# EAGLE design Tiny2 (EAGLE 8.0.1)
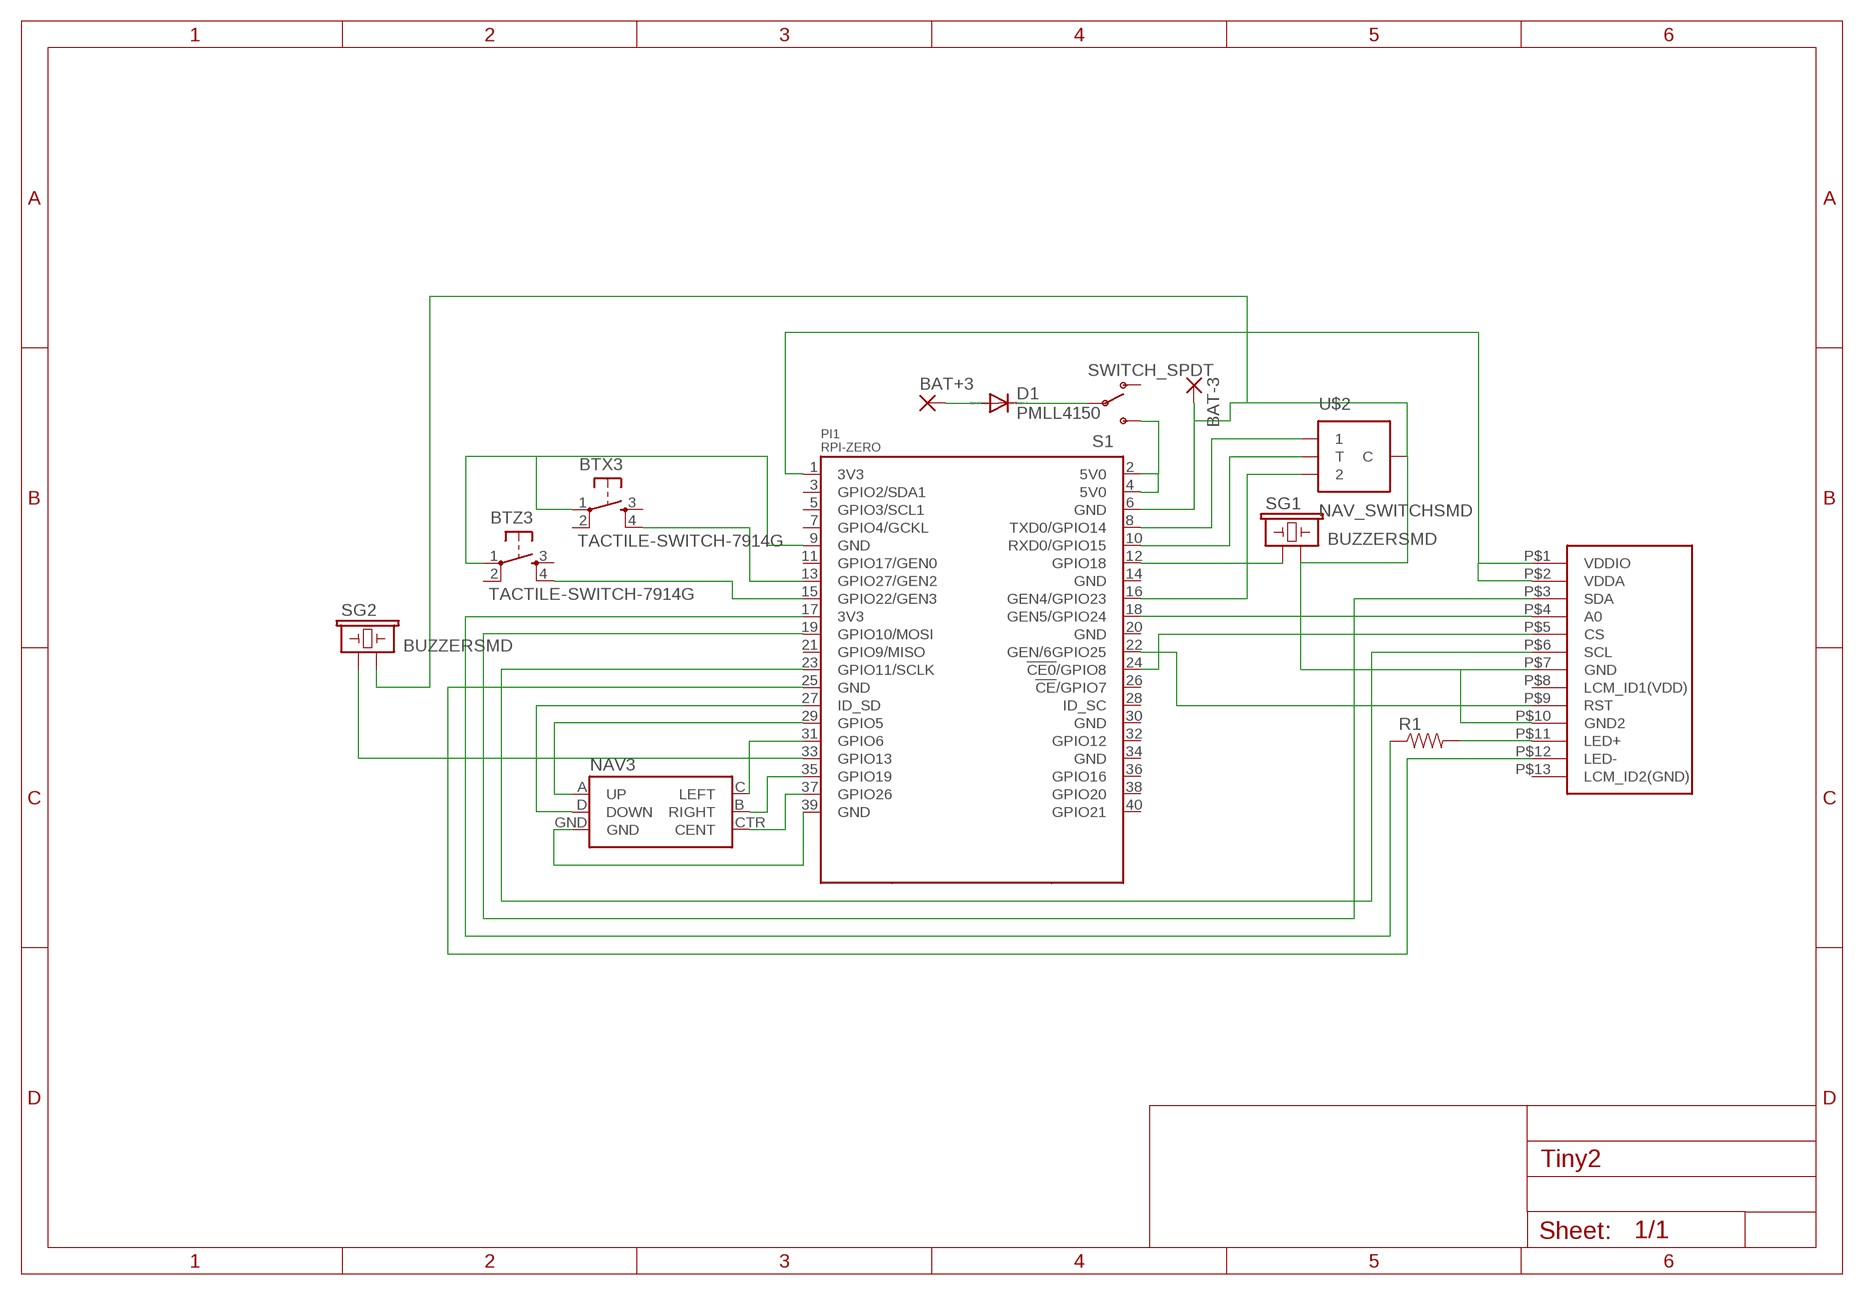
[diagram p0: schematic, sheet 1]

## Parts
BAT+3  SMD5  [SMD2,54-5,08]
BAT-3  SMD5  [SMD2,54-5,08]
BTX3  TACTILE-SWITCH-7914G  [7914G]
BTZ3  TACTILE-SWITCH-7914G  [7914G]
D1  PMLL4150  [SOD80C]
NAV3  JOYSTICK_MINI  [JOYSTICK_MINI]
PI1  RPI-ZERO  [RASPBERRYPI_BASTELSTUBE_V13_RASPI_BOARD_B+_FULL]
R1  RESISTOR0805-RES  [0805]
S1  SWITCH_SPDT  [KPS-1290]
SG1  BUZZERSMD  [BUZZER-CMT1603]
SG2  BUZZERSMD  [BUZZER-CMT1603]
U$1  ST7735S-1.44  [ST7735S-1.44]
U$2  NAV_SWITCHSMD  [NAV_SWITCH]

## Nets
3V3@1: PI1.1(3V3) U$1.P$1(VDDIO) U$1.P$2(VDDA)
3V3@2: PI1.17(3V3) R1.1
5V0@2: PI1.2(5V0) PI1.4(5V0) S1.S
GND@1: BTX3.1 BTZ3.1 PI1.9(GND)
GND@2: PI1.25(GND) U$1.P$12(LED-)
GND@3: NAV3.GND PI1.39(GND)
GND@8: BAT-3.1(P) PI1.6(GND) SG1.P$2 SG2.P$2 U$1.P$7(GND) U$1.P$10(GND2) U$2.C
N$1: PI1.22(GEN/6GPIO25) U$1.P$9(RST)
N$2: PI1.23(GPIO11/SCLK) U$1.P$6(SCL)
N$3: PI1.19(GPIO10/MOSI) U$1.P$3(SDA)
N$4: NAV3.CTR(CENT) PI1.37(GPIO26)
N$5: NAV3.B(RIGHT) PI1.35(GPIO19)
N$6: PI1.18(GEN5/GPIO24) U$1.P$4(A0)
N$7: PI1.24(!CE0!/GPIO8) U$1.P$5(CS)
N$8: NAV3.C(LEFT) PI1.31(GPIO6)
N$9: NAV3.A(UP) PI1.29(GPIO5)
N$10: NAV3.D(DOWN) PI1.27(ID_SD)
N$11: BTZ3.4 PI1.15(GPIO22/GEN3)
N$12: BTX3.4 PI1.13(GPIO27/GEN2)
N$13: PI1.12(GPIO18) SG1.P$1
N$14: R1.2 U$1.P$11(LED+)
N$15: PI1.33(GPIO13) SG2.P$1
N$16: PI1.8(TXD0/GPIO14) U$2.1
N$17: PI1.10(RXD0/GPIO15) U$2.T
N$18: PI1.16(GEN4/GPIO23) U$2.2
N$20: BAT+3.1(P) D1.A
N$21: D1.C S1.P
Unconnected: BTX3.2 BTX3.3 BTZ3.2 BTZ3.3 PI1.3(GPIO2/SDA1) PI1.5(GPIO3/SCL1) PI1.7(GPIO4/GCKL) PI1.11(GPIO17/GEN0) PI1.14(GND) PI1.20(GND) PI1.21(GPIO9/MISO) PI1.26(!CE!/GPIO7) PI1.28(ID_SC) PI1.30(GND) PI1.32(GPIO12) PI1.34(GND) PI1.36(GPIO16) PI1.38(GPIO20) PI1.40(GPIO21) S1.O U$1.P$8(LCM_ID1(VDD)) U$1.P$13(LCM_ID2(GND))

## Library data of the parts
BAT+3 BAT-3 = wirepad:SMD5: SMD PAD
BTX3 BTZ3 = GeekAmmo:TACTILE-SWITCH: Tactile Switch 4 Pins, SPST NO
D1 = diode:PMLL4150: DIODE
NAV3 = SparkFun-Electromechanical:JOYSTICK_MINI: Small 5-way tactile joystick, COM-10063 4UCON SF303GJ26; PROD_ID: SWCH-09905
PI1 = RPI-Zero:RPI-ZERO
R1 = SparkFun-Resistors:RESISTOR: Resistor
S1 = SparkFun-Electromechanical:SWITCH_SPDT: SWCH-10651 Side-actuated SPDT slide switch, as used on the Arduino Pro; PROD_ID: SWCH-10651
SG1 SG2 = SparkFun-Electromechanical:BUZZER: Buzzer 12mm
U$1 = ST7735S:ST7735S-1.44
U$2 = SparkFun-Electromechanical:NAV_SWITCH: Navigation Switch Three way navigation switch. Commonly used as up/down/select on MP3 players. Schematic element and footprint production proven. Spark Fun Electronics SKU : COM-08184; PROD_ID: SWCH-08301

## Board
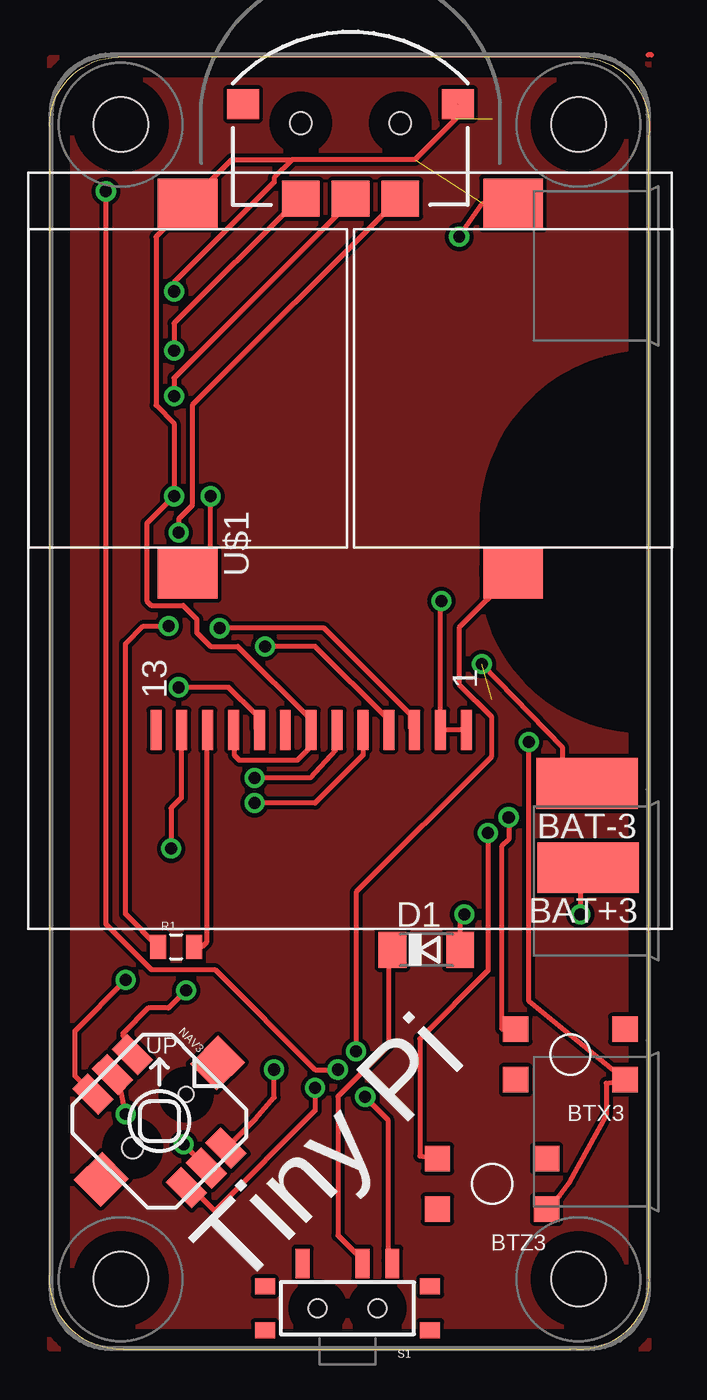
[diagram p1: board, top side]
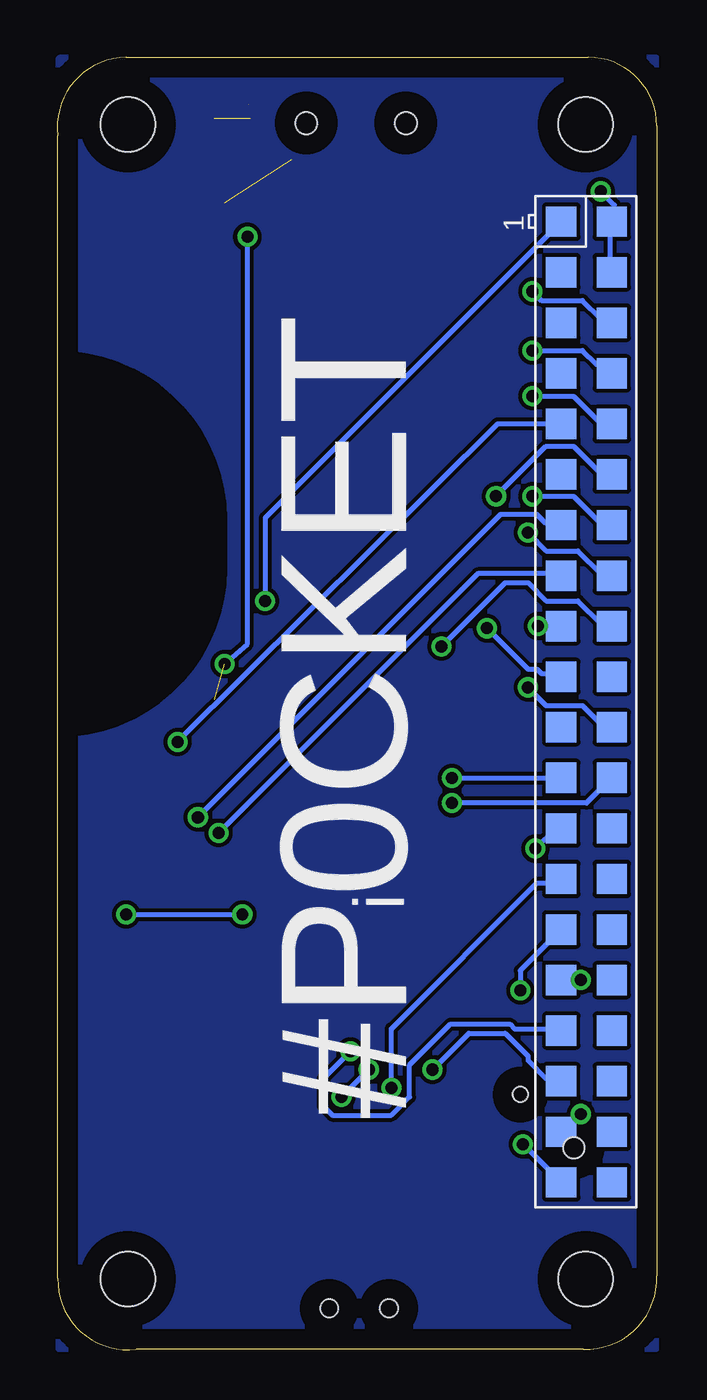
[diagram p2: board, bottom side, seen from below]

Size 30.12 x 64.92 mm. Coordinates in mm from the lower left corner, seen from the top.
Outline: 3.68,0.03 26.16,0.03 arc98 30.1,3.58 30.1,60.99 arc96 26.67,64.92 3.43,64.92 arc90 0,61.49 0,3.71 arc94 3.68,0.03
Copper layers (1*16): Top 0.035mm / dielectric 1.5mm / Bottom 0.035mm
Design rules "default *": minimum track width 10mil, minimum drill 24mil, track to track 8mil, track to pad 8mil, pad to pad 8mil, via to via 8mil, smd to smd 8mil, copper to edge 40mil, drill to drill 8mil, minimum pad ring 10mil, minimum via ring 8mil, stop-mask expansion 4mil, vias tented up to drill 25mil, thermal gap 10mil

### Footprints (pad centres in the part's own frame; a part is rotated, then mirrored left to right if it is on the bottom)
SMD2,54-5,08 = smd 2.54 x 5.08: 1 0,0
7914G = smd 1.27 x 1.27: 1 0,0; 2 0,5.486; 3 2.54,0; 4 2.54,5.486
SOD80C = smd 1.4 x 1.8: A 1.7,0; C -1.7,0
JOYSTICK_MINI = smd 1.85 x 1.1: A -3.325,1.4; B 3.325,1.4; C -3.325,-1.4; CTR -3.325,0; D 3.325,-1.4; GND 3.325,0 | smd 1.9 x 2: NC 0,4.13; NC@0 0,-4.13 | hole 0.75: 0,1.9 | hole 1.05: 0,-1.9
RASPBERRYPI_BASTELSTUBE_V13_RASPI_BOARD_B+_FULL = smd 1.524 x 1.524: 1 8.382,25.273; 2 8.382,27.813; 3 10.922,25.273; 4 10.922,27.813; 5 13.462,25.273; 6 13.462,27.813; 7 16.002,25.273; 8 16.002,27.813; 9 18.542,25.273; 10 18.542,27.813; 11 21.082,25.273; 12 21.082,27.813; 13 23.622,25.273; 14 23.622,27.813; 15 26.162,25.273; 16 26.162,27.813; 17 28.702,25.273; 18 28.702,27.813; 19 31.242,25.273; 20 31.242,27.813; 21 33.782,25.273; 22 33.782,27.813; 23 36.322,25.273; 24 36.322,27.813; 25 38.862,25.273; 26 38.862,27.813; 27 41.402,25.273; 28 41.402,27.813; 29 43.942,25.273; 30 43.942,27.813; 31 46.482,25.273; 32 46.482,27.813; 33 49.022,25.273; 34 49.022,27.813; 35 51.562,25.273; 36 51.562,27.813; 37 54.102,25.273; 38 54.102,27.813; 39 56.642,25.273; 40 56.642,27.813 | hole 2.75: 3.5,3.5; 3.5,26.5; 61.5,3.5; 61.5,26.5
0805 = smd 0.8 x 1.2: 1 -0.9,0; 2 0.9,0
KPS-1290 = smd 0.7 x 1.5: O -2.25,2.25; P 0.75,2.25; S 2.25,2.25 | smd 1 x 0.8: P$1 -4.15,1.1; P$2 -4.15,-1.1; P$3 4.15,-1.1; P$4 4.15,1.1 | hole 0.9: -1.5,0; 1.5,0
BUZZER-CMT1603 = smd 2.5 x 3: P$1 -9.3,0; P$2 9.3,0
ST7735S-1.44 = smd 2 x 0.55: P$1 -9,-5.85; P$2 -9,-4.55; P$3 -9,-3.25; P$4 -9,-1.95; P$5 -9,-0.65; P$6 -9,0.65; P$7 -9,1.95; P$8 -9,3.25; P$9 -9,4.55; P$10 -9,5.85; P$11 -9,7.15; P$12 -9,8.45; P$13 -9,9.75
NAV_SWITCH = smd 1.9 x 1.8: 1 -2.5,-3.8; 2 2.5,-3.8; T 0,-3.8 | smd 1.6 x 1.5: C 5.4,0.95; NC -5.4,0.95 | hole 1.1: -2.5,0; 2.5,0

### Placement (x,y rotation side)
BAT+3  27.05,24.21 90 top
BAT-3  27,28.45 90 top
BTX3  28.91,13.56 90 top
BTZ3  24.97,7.06 90 top
D1  18.92,20.09 0 top
NAV3  5.51,11.48 315 top
PI1  30.07,65.05 270 bottom
R1  6.35,20.24 0 top
S1  14.96,2.08 0 top
SG1  6.93,48.29 90 top
SG2  23.29,48.29 90 top
U$1  15.09,40.13 90 top
U$2  15.11,61.62 0 top

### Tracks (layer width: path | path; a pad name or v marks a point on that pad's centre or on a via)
3V3@1  (via drill 0.6)
  Top 0.254: v19.69,37.62 19.64,37.57 U$1.P$2 U$1.P$1
  Bottom 0.254: PI1.1 19.69,41.78 v19.69,37.62
3V3@2  (via drill 0.6)
  Top 0.254: R1.1 3.81,21.88 3.81,35.46 4.7,36.35 v5.97,36.35
  Bottom 0.254: v5.97,36.35 PI1.17
5V0@2  (via drill 0.61)
  Top 0.254: v15.85,12.7 16.99,11.56 16.99,4.47 S1.S | v14.48,14.07 13.33,14.07 8.31,19.1 5.11,19.1 2.82,21.39 v2.82,58.19
  Bottom 0.254: v14.48,14.07 v15.85,12.7 | v2.82,58.19 2.13,57.51 2.13,56.82 PI1.2 2.36,56.59 2.36,54.31 PI1.4
GND@1  (via drill 0.61)
  Top 0.254: BTZ3.1 25.6,7.72 26.11,8.41 27.97,11.79 27.97,13.39 BTX3.1 24.08,17.5 v24.08,30.53
  Bottom 0.254: 4.88,46.53 PI1.9 8,46.51 23.9,30.73 | 23.9,30.73 24.08,30.43 | v24.08,30.53 23.9,30.73
GND@2  (via drill 0.6)
  Top 0.254: U$1.P$12 6.6,31.1 6.6,27.71 6.1,27.2 v6.1,25.17
  Bottom 0.254: v6.1,25.17 5.08,26.19 PI1.25
GND@3  (via drill 0.6)
  Top 0.254: v6.73,10.31 7.86,9.18 NAV3.GND
  Bottom 0.254: PI1.39 6.71,10.31 v6.73,10.31
GND@8  (via drill 0.6, 0.61)  (4 unrouted)
  Top 0.254: v6.25,53.16 6.25,53.62 11.28,58.65 11.28,58.88 12.19,59.79 | 12.19,59.79 18.36,59.79 20.42,61.85 | 20.42,61.85 20.42,62.53 U$2.C 20.42,61.85 | 12.19,59.79 9.14,59.79 SG1.P$2 6.93,57.51 5.33,55.91 5.33,47.45 6.25,46.53 v6.25,42.88 4.88,41.5 4.88,37.62 5.11,37.39 6.71,37.39 7.39,36.7 7.39,36.02 8.08,35.33 9.45,35.33 13.11,31.67 13.11,31.22 U$1.P$7 13.14,30.31 12.45,29.62 9.53,29.62 9.27,29.87 9.27,31.1 U$1.P$10 | 23.39,57.68 SG2.P$2 21.75,57.59 v20.57,55.91 | BAT-3.1 25.78,29.67 25.78,30.25 v21.72,34.44
  Bottom 0.254: v6.25,53.16 5.79,52.71 3.73,52.71 2.82,51.79 2.36,51.79 PI1.6 | 2.36,41.5 2.82,41.5 4.19,42.88 v6.25,42.88 | v21.72,34.44 20.57,35.46 v20.57,55.91
N$1  (via drill 0.61)
  Top 0.254: v6.48,33.27 8.99,33.27 10.36,31.9 10.36,31.22 U$1.P$9
  Bottom 0.254: v6.48,33.27 5.56,32.36 3.73,32.36 2.82,31.45 2.36,31.45 PI1.22
N$2  (via drill 0.6)
  Top 0.254: U$1.P$6 14.35,31.05 14.35,30.12 13.08,28.73 v10.29,28.73
  Bottom 0.254: v10.29,28.73 PI1.23
N$3  (via drill 0.61)
  Top 0.254: v8.53,36.25 13.79,36.25 18.14,31.9 18.14,31.22 U$1.P$3
  Bottom 0.254: v8.53,36.25 6.48,34.19 6.02,34.19 5.79,33.96 4.88,33.96 PI1.19
N$4  (via drill 0.6)
  Top 0.254: v3.81,11.84 3.56,13.11 3.21,13.83 NAV3.CTR
  Bottom 0.254: PI1.37 3.81,11.81 v3.81,11.84
N$5  (via drill 0.61)
  Top 0.254: v11.28,14.07 11.28,12.67 10.34,11.61 NAV3.B
  Bottom 0.254: v11.28,14.07 9.45,15.9 7.62,15.9 6.48,14.76 6.48,14.53 5.56,13.61 4.88,13.61 PI1.35
N$6  (via drill 0.61)
  Top 0.254: v10.82,35.33 13.33,35.33 16.99,31.67 16.99,31.22 U$1.P$4
  Bottom 0.254: v10.82,35.33 7.62,38.53 6.48,38.53 5.56,37.62 3.96,37.62 2.82,36.47 2.36,36.47 PI1.18
N$7  (via drill 0.6)
  Top 0.254: U$1.P$5 15.75,31.12 15.75,29.87 13.33,27.46 v10.29,27.46
  Bottom 0.254: PI1.24 3.53,27.46 v10.29,27.46
N$8  (via drill 0.6)
  Top 0.254: NAV3.C 1.27,13.74 1.27,16.03 v3.81,18.57
  Bottom 0.254: v3.81,18.57 PI1.31
N$9  (via drill 0.6)
  Top 0.254: v6.86,18.06 5.97,17.17 4.95,17.17 3.68,15.9 3.68,15.77 4.15,15.31 NAV3.A
  Bottom 0.254: PI1.29 6.86,19.05 v6.86,18.06
N$10  (via drill 0.61)
  Top 0.254: v13.33,13.16 13.33,12.01 8.33,7.01 8.26,7.01 7.13,8.14 NAV3.D
  Bottom 0.254: v13.33,13.16 13.33,16.13 6.02,23.44 4.88,23.44 PI1.27
N$11  (via drill 0.61)
  Top 0.254: v22.02,25.96 22.02,19.05 18.59,15.62 18.59,9.73 BTZ3.4
  Bottom 0.254: v22.02,25.96 8.99,38.99 4.88,38.99 PI1.15
N$12  (via drill 0.61)
  Top 0.254: v23.06,26.75 23.06,25.63 22.71,25.27 22.71,16.13 BTX3.4
  Bottom 0.254: v23.06,26.75 7.85,41.96 6.02,41.96 5.56,41.5 4.88,41.5 PI1.13
N$13  (via drill 0.61)
  Top 0.254: v8.08,42.88 8.08,40.13 SG1.P$1
  Bottom 0.254: v8.08,42.88 5.56,45.39 4.19,45.39 2.82,44.02 2.36,44.02 PI1.12
N$14
  Top 0.254: U$1.P$11 7.87,31.07 7.87,20.47 7.64,20.24 R1.2
N$15  (via drill 0.61)
  Top 0.254: v15.39,14.99 15.39,22.99 22.19,29.78 22.19,31.81 20.57,33.43 20.57,36.27 SG2.P$1 23.16,38.76
  Bottom 0.254: v15.39,14.99 16.76,13.61 16.76,12.24 16.31,11.79 13.33,11.79 12.42,12.7 12.42,14.3 10.36,16.36 7.39,16.36 7.16,16.13 4.88,16.13 PI1.33
N$16  (via drill 0.61)
  Top 0.254: v6.25,50.19 6.25,51.56 12.42,57.73 U$2.1
  Bottom 0.254: v6.25,50.19 3.73,50.19 3.05,49.5 2.82,49.5 2.36,49.05 PI1.8
N$17  (via drill 0.61)
  Top 0.254: v6.25,47.9 6.25,48.82 15.16,57.73 U$2.T
  Bottom 0.254: v6.25,47.9 4.19,47.9 2.82,46.53 2.36,46.53 PI1.10
N$18  (via drill 0.61)
  Top 0.254: v6.48,41.05 6.48,41.73 7.16,42.42 7.16,47.45 17.45,57.73 U$2.2
  Bottom 0.254: v6.48,41.05 5.56,40.13 3.96,40.13 2.82,38.99 2.36,38.99 PI1.16
N$19
  pour Bottom: 30.1,50.32 arc90 21.46,41.68 21.46,39.27 arc90 30.1,30.63 30.1,0.03 0,0.03 0,64.92 29.97,64.92 arc-90 30.1,64.8
N$20  (via drill 0.6)
  Top 0.254: BAT+3.1 26.67,23.83 v26.67,21.87 | v20.83,21.87 20.62,21.66 D1.A
  Bottom 0.254: v26.67,21.87 v20.83,21.87
N$21
  Top 0.254: D1.C 17.02,19.38 17.02,15.27 14.48,12.73 14.48,5.74 15.71,4.51 S1.P
N$22
  Top 0.254: 30.25,65.05 30.07,65.05
N$25
  pour Top: 30.1,50.32 arc90 21.46,41.68 21.46,39.78 arc90 29.21,30.89 30.1,30.63 30.1,0.03 0,0.03 0,64.92 30.1,64.92

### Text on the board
tNames: Tiny Pi
bNames: i | #P0CKET
UNCONECTED_WireText: TE:N$22:4:4::L1 | TS:N$22:4:4::L1 | TS:GND@8:1:4::L19 | TE:GND@8:1:4::L19 | TS:GND@8:3:4::L19 | TE:GND@8:3:4::L19 | TE:GND@8:2:4::L19 | TS:GND@8:2:4::L19

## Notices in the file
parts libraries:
SparkFun-Electromechanical: Licensing: Creative Commons ShareAlike 4.0 International - https://creativecommons.org/licenses/by-sa/4.0
